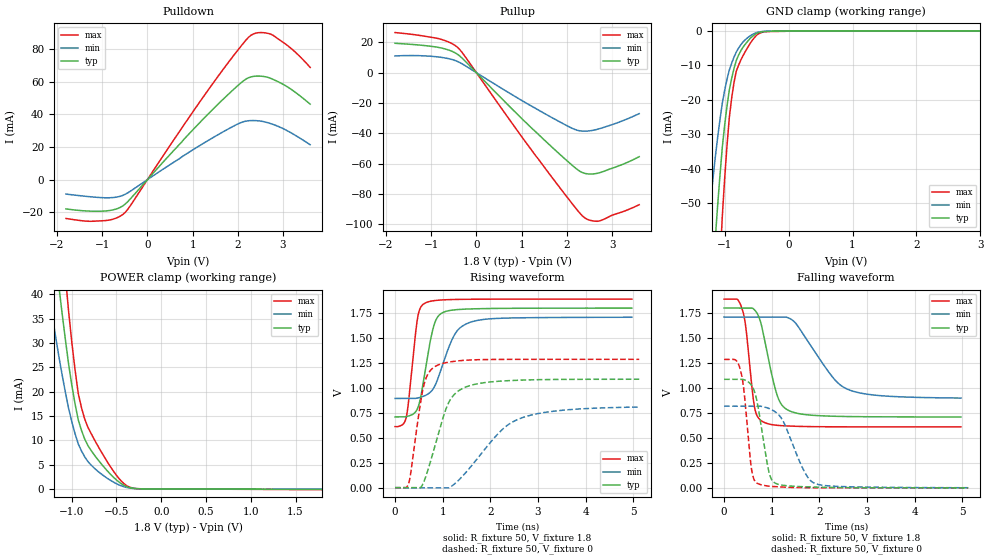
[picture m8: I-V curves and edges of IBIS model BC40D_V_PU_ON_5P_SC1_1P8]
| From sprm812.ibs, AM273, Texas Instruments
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|   Model Cell BC40D_V_PU_ON_5P_SC1_1P8
|BC40D_V_PU_ON_5P_SC1_1P8
[Model]   BC40D_V_PU_ON_5P_SC1_1P8
Model_type   I/O
Polarity   Non-Inverting
Enable   Active-Low
Vinl =  0.63
Vinh =  1.17
Cref =  15pF
Rref =  100.0000M
Vref =  0V
Vmeas =  0.9
C_comp   2.233931p   2.204415p   2.290246p
|[Input load] weak_pu_on
|[Output drive] slow
|[supplytol] 5
|[temp] ind
[Model Spec]
Vinl   0.63   0.5985   0.6615
Vinh   1.17   1.1115   1.2285
[Temperature Range]   25   125   -40
[Voltage Range]   1.8   1.71   1.89
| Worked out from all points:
|   slope of the pulldown table from 0 to 0.27 V, typ, clamps not added: 32.2 ohm
|   slope of the pullup table from 0 to 0.27 V, typ, clamps not added: 32.6 ohm
|   GND clamp passes 1 mA (typ) near -0.52 V on its own axis
|   POWER clamp passes 1 mA (typ) near -0.44 V on its own axis
|   rising waveform, R_fixture 50, V_fixture 1.8: 20-80 % time 245ps typ, 395ps min, 168ps max; typ from 0.711 V to 1.8 V
|   rising waveform, R_fixture 50, V_fixture 0: 20-80 % time 428ps typ, 921ps min, 245ps max; typ from 0.002 V to 1.09 V
|   falling waveform, R_fixture 50, V_fixture 1.8: 20-80 % time 308ps typ, 718ps min, 171ps max; typ from 1.8 V to 0.71 V
|   falling waveform, R_fixture 50, V_fixture 0: 20-80 % time 226ps typ, 430ps min, 154ps max; typ from 1.09 V to 0.002 V
| Nom Voltages:
|   VDD=1.1, VDDS=1.8, VDDS18=1.8, ESD_BIASFET=0, VSS=0, VSSS=0
| Min Voltages:
|   VDD=1.045, VDDS=1.71, VDDS18=1.71, ESD_BIASFET=0, VSS=0, VSSS=0
| Max Voltages:
|   VDD=1.16, VDDS=1.89, VDDS18=1.89, ESD_BIASFET=0, VSS=0, VSSS=0
[POWER_clamp]
|   voltage   I(typ)   I(min)   I(max)
-1.8V     158.8mA    112.5mA    219.8mA
-1.255V   59.97mA    40.01mA    84.91mA
-1.145V   41.92mA    27.41mA    59.76mA
-1.109V   36.32mA    23.62mA    51.83mA
-1.073V   30.96mA    20.04mA    44.16mA
-1.036V   25.83mA    16.67mA    36.76mA
-963.6mV  17.54mA    11.39mA    24.56mA
-890.9mV  12.01mA    7.798mA    16.67mA
-818.2mV  8.875mA    5.598mA    12.64mA
-563.6mV  2.954mA    1.726mA    4.46mA
-272.7mV  55.97uA    39.54uA    57.56uA
1.8V      -99.94uA   -59.14uA   -145.1uA
[Pulldown]
|   voltage   I(typ)   I(min)   I(max)
-1.8V     -17.92mA   -8.85mA    -23.8mA
-1.309V   -19.26mA   -10.37mA   -25.51mA
-927.3mV  -19.22mA   -11.12mA   -25.08mA
-654.5mV  -17.65mA   -10.56mA   -23.13mA
-490.9mV  -14.97mA   -8.985mA   -20.05mA
1.364V    40.78mA    24.32mA    55.7mA
2.073V    59.41mA    35mA       81.9mA
2.291V    62.96mA    36.2mA     88.48mA
2.509V    63.41mA    35.84mA    90.12mA
2.782V    61.38mA    33.82mA    88.42mA
3.218V    54.59mA    28.02mA    79.45mA
3.6V      46.26mA    21.39mA    68.79mA
[Pullup]
|   voltage   I(typ)   I(min)   I(max)
-1.8V     19.42mA    11.07mA    26.5mA
-818.2mV  16.58mA    10.3mA     22.34mA
-545.5mV  14.19mA    8.748mA    19.29mA
-381.8mV  11.34mA    6.915mA    15.7mA
1.255V    -37.51mA   -22.64mA   -52.53mA
2.127V    -61.34mA   -36.82mA   -86.78mA
2.291V    -65.12mA   -38.38mA   -92.82mA
2.4V      -66.46mA   -38.59mA   -95.91mA
2.564V    -66.86mA   -38.08mA   -97.75mA
2.727V    -65.99mA   -36.9mA    -97.78mA
3.273V    -60.01mA   -31.26mA   -91.34mA
3.6V      -55.4mA    -26.98mA   -87.12mA
[GND_clamp]
|   voltage   I(typ)   I(min)   I(max)
-1.8V     -270.2mA   -170.2mA   -430.1mA
-1.255V   -91.68mA   -55.92mA   -148.5mA
-1.145V   -59.94mA   -36.46mA   -97.14mA
-1.109V   -50.51mA   -30.84mA   -81.61mA
-1.073V   -41.77mA   -25.67mA   -67.13mA
-1.036V   -33.71mA   -20.95mA   -53.68mA
-927.3mV  -17.15mA   -11.38mA   -25.19mA
-854.5mV  -10.96mA   -7.663mA   -15.08mA
-781.8mV  -7.031mA   -5.001mA   -9.947mA
-563.6mV  -1.569mA   -1.041mA   -2.641mA
-18.18mV  0A         0A         0A
3.6V      0A         0A         0A
[Ramp]
| variable   typ   min   max
dV/dt_f 0.66095896/0.3106084n 0.49613312/0.73326127n 0.77259659/0.17250259n
dV/dt_r 0.65862655/0.43190461n 0.50230725/0.96092972n 0.77696157/0.24571965n
R_load = 50
[Rising Waveform]
R_fixture = 50
V_fixture = 1.8
V_fixture_min = 1.71
V_fixture_max = 1.89
|   time   V(typ)   V(min)   V(max)
0s        710.6mV    895.2mV    613.1mV
234.7ps   712.8mV    895.2mV    706mV
279.7ps   718.7mV    895.2mV    848.3mV
472.8ps   795.2mV    899.6mV    1.7V
625.3ps   1.154V     923mV      1.849V
773.2ps   1.547V     974.1mV    1.871V
891.9ps   1.709V     1.084V     1.879V
1.246ns   1.783V     1.53V      1.887V
1.553ns   1.791V     1.654V     1.889V
4.974ns   1.8V       1.708V     1.89V
[Rising Waveform]
R_fixture = 50
V_fixture = 0
V_fixture_min = 0
V_fixture_max = 0
|   time   V(typ)   V(min)   V(max)
0s        2.021mV    0V         2.349mV
286.7ps   2.021mV    0V         46.67mV
600.6ps   55.49mV    0V         1.02V
705.3ps   201.5mV    0V         1.151V
868.1ps   473.5mV    0V         1.223V
1.162ns   884.2mV    8.941mV    1.262V
1.566ns   1.023V     197.8mV    1.28V
2.228ns   1.069V     573.6mV    1.286V
2.667ns   1.079V     702.1mV    1.287V
5.128ns   1.088V     808.9mV    1.287V
[Falling Waveform]
R_fixture = 50
V_fixture = 1.8
V_fixture_min = 1.71
V_fixture_max = 1.89
|   time   V(typ)   V(min)   V(max)
0s        1.8V       1.71V      1.889V
275ps     1.8V       1.71V      1.889V
378.3ps   1.8V       1.71V      1.793V
458.3ps   1.8V       1.71V      1.601V
639.6ps   1.782V     1.71V      809mV
817.4ps   1.559V     1.71V      662.6mV
1.117ns   924.9mV    1.71V      627.2mV
1.374ns   771.8mV    1.697V     619.7mV
2.563ns   715.4mV    994.7mV    612.1mV
4.974ns   710.1mV    900mV      611.7mV
[Falling Waveform]
R_fixture = 50
V_fixture = 0
V_fixture_min = 0
V_fixture_max = 0
|   time   V(typ)   V(min)   V(max)
0s        1.087V     818.9mV    1.286V
342.4ps   1.087V     818.9mV    1.183V
418.5ps   1.083V     818.9mV    970.8mV
572.8ps   1.03V      818.9mV    201.5mV
701.2ps   844.1mV    818.9mV    46.7mV
936.2ps   172.9mV    797.1mV    19.49mV
1.095ns   44.58mV    755.1mV    13.55mV
1.708ns   12.56mV    145.8mV    3.939mV
1.914ns   10.01mV    45.38mV    3.232mV
5.128ns   2.074mV    3.413mV    2.43mV
